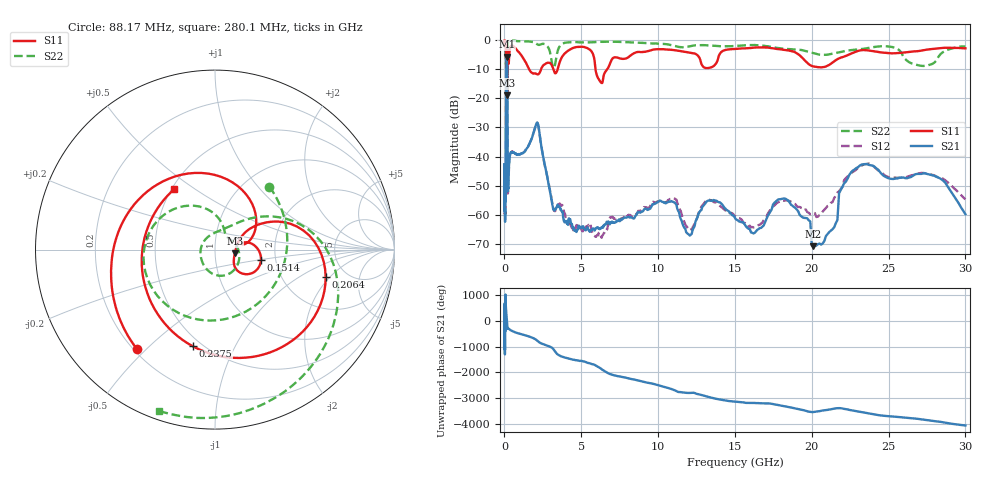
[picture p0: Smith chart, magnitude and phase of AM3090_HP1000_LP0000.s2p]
! Date/Time: Thu, Feb 28, 2019 2:01 PM
! Network Analyzer: Agilent Technologies E8364B Rev: A.07.50.67
! Sweep from 0.010 to 30.000 GHz, 1601 Points, Sweep Type: LOG
! Power Supply: 5.023 V, 0.002 A
# Hz S DB R 50
!freq MagS11 AngS11 MagS21 AngS21 MagS12 AngS12 MagS22 AngS22
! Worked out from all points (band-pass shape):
!   1601 points, 10 MHz to 30 GHz, reference 50 ohm
!   highest |S21| = -5.70 dB at 142.6 MHz (marker M1); lowest = -70.8 dB at 20.1 GHz (marker M2)
!   |S21| within 3 dB of the highest: 120.8 MHz to 176.9 MHz (56.01 MHz wide, 37.6 % of centre)
!   lowest |S11| = -19.0 dB at 179.4 MHz (marker M3), VSWR 1.25, Z = 62.4 - j2.49 ohm
!   |S11| at or under -10 dB: 1.604 GHz to 2.384 GHz (779.5 MHz wide, 39.1 % of centre); 3.183 GHz to 3.465 GHz (282 MHz wide, 8.49 % of centre); 5.925 GHz to 6.694 GHz (768.9 MHz wide, 12.2 % of centre)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
!   |S22| runs from -22.3 to -0.1 dB; largest |S21 - S12| = 0.014
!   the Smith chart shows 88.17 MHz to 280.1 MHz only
!   S11 on the Smith chart (normalised r, x): 88.17 MHz: 0.21, -0.47; 151.4 MHz: 1.67, -0.20; 206.4 MHz: 3.52, -1.78; 237.5 MHz: 0.45, -0.69; 280.1 MHz: 0.52, +0.42
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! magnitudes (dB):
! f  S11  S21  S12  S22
! 10 MHz  -0.2  -42.7  -42.4  -0.5
! 38.04 MHz  -0.5  -59.7  -58.4  -1.2
! 48.61 MHz  -0.8  -47.4  -51.5  -1.4
! 88.17 MHz  -3.0  -49.2  -49.3  -6.7
! 116.7 MHz  -8.8  -11.4  -11.4  -9.8
! 142.6 MHz  -13.2  -5.7  -5.7  -17.8
! 144.7 MHz  -12.6  -5.7  -5.7  -17.2
! 151.4 MHz  -11.6  -5.8  -5.8  -16.1
! 179.4 MHz  -19.0  -9.7  -9.6  -18.4
! 206.4 MHz  -3.9  -47.9  -47.8  -2.5
! 237.5 MHz  -5.2  -51.2  -51.9  -0.8
! 280.1 MHz  -7.8  -45.2  -45.6  -0.4
! 550.5 MHz  -2.1  -38.5  -38.4  -0.2
! 2.084 GHz  -11.6  -28.7  -28.6  -1.3
! 3.22 GHz  -10.6  -58.4  -58.5  -9.6
! 7.926 GHz  -6.3  -61.0  -60.5  -0.7
! 13.61 GHz  -9.0  -54.9  -55.6  -1.9
! 16.29 GHz  -2.6  -66.2  -64.3  -1.7
! 18.19 GHz  -3.4  -54.4  -55.2  -3.0
! 20.1 GHz  -9.1  -70.8  -59.4  -4.5
! 23.36 GHz  -3.4  -42.7  -42.8  -3.0
! 30 GHz  -2.8  -59.8  -54.7  -2.2
